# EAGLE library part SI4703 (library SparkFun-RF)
Silicon Labs Si4703 FM Tuner Beyond enabling you to tune in to FM radio stations, the Si4703 is also capable of detecting and processing both Radio Data Service (RDS) and Radio Broadcast Data Service (RBDS) information. The Si4703 even does a very good job of filtering and carrier detection. It also enables data such as the station ID and song name to be displayed to the user. SparkFun Products SparkFun FM Tuner Evaluation Board - Si4703 (WRL-12938) SparkFun FM Tuner Basic Breakout - Si4703 (WRL-11083) FabFM Radio Kit (KIT-11043)
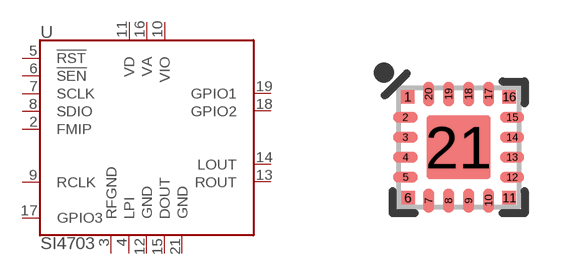
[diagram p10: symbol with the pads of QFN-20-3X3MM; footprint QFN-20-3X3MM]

Designator prefix U

## SI4703 (PROD_ID: IC-10150)  [QFN-20-3X3MM]
2  FMIP
3  RFGND
4  LPI
5  !RST
6  !SEN
7  SCLK
8  SDIO
9  RCLK
10  VIO
11  VD
12  GND
13  ROUT
14  LOUT
15  DOUT
16  VA
17  GPIO3
18  GPIO2
19  GPIO1
21  GND

## Footprint QFN-20-3X3MM (pad centres in mm)
20-Pin QFN Package 3 x 3 mm Used by Silicon Labs Si470x (Si4703, Si4707, etc.) FM Recievier Example Datasheet
smd 0.34 x 0.34: 1 -1.275,1.265; 6 -1.265,-1.265; 11 1.265,-1.265; 16 1.265,1.265
smd 0.61 x 0.28: 2 -1.335,0.75; 3 -1.335,0.25; 4 -1.335,-0.25; 5 -1.335,-0.75; 12 1.335,-0.75; 13 1.335,-0.25; 14 1.335,0.25; 15 1.335,0.75
smd 0.28 x 0.61: 7 -0.75,-1.335; 8 -0.25,-1.335; 9 0.25,-1.335; 10 0.75,-1.335; 17 0.75,1.335; 18 0.25,1.335; 19 -0.25,1.335; 20 -0.75,1.335
smd 1.6 x 1.6: 21 0,0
